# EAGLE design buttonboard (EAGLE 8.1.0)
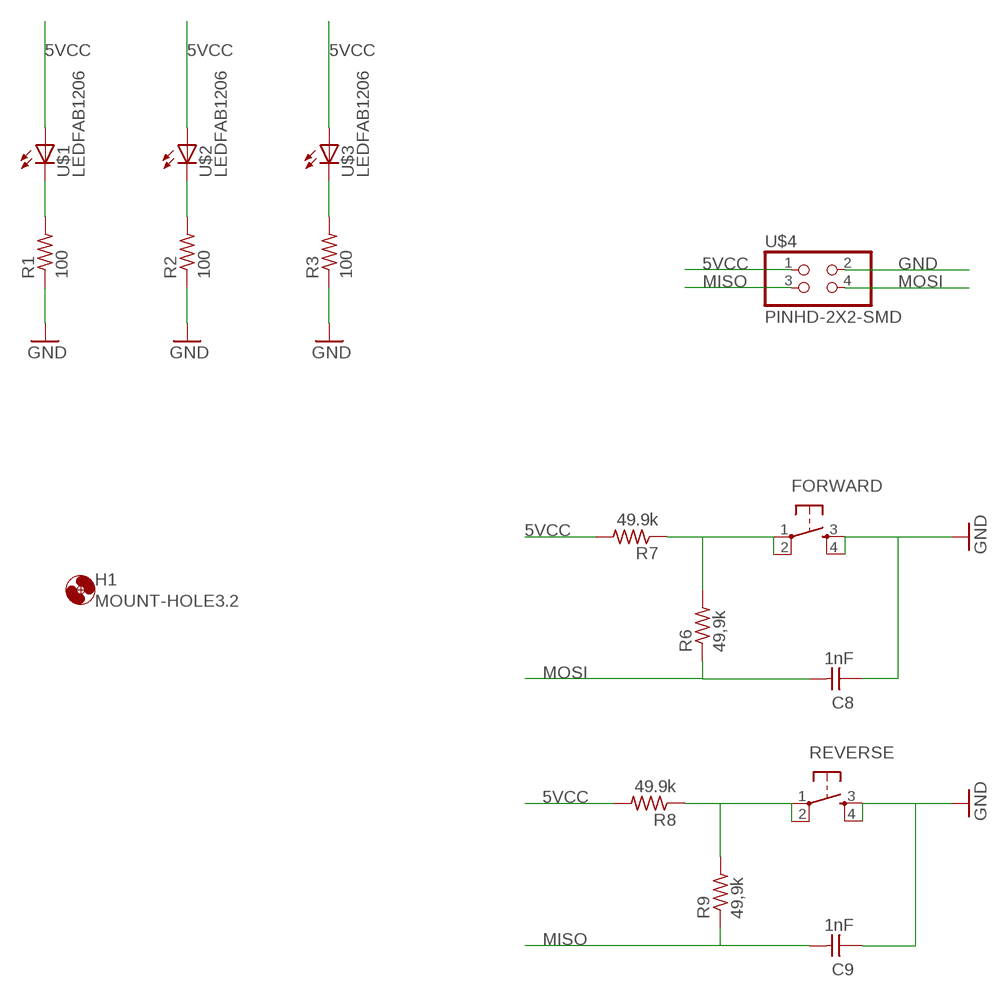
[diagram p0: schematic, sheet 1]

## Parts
C8  1nF  CAP-UNPOLARIZEDFAB  [C1206FAB]
C9  1nF  CAP-UNPOLARIZEDFAB  [C1206FAB]
FORWARD  6MM_SWITCH6MM_SWITCH  [6MM_SWITCH]
H1  MOUNT-HOLE3.2  [3,2]
R1  100  RES-US1206FAB  [R1206FAB]
R2  100  RES-US1206FAB  [R1206FAB]
R3  100  RES-US1206FAB  [R1206FAB]
R6  49,9k  RES-US1206FAB  [R1206FAB]
R7  49.9k  RES-US1206FAB  [R1206FAB]
R8  49.9k  RES-US1206FAB  [R1206FAB]
R9  49,9k  RES-US1206FAB  [R1206FAB]
REVERSE  6MM_SWITCH6MM_SWITCH  [6MM_SWITCH]
U$1  LEDFAB1206  [LED1206FAB]
U$2  LEDFAB1206  [LED1206FAB]
U$3  LEDFAB1206  [LED1206FAB]
U$4  PINHD-2X2-SMD  [2X02SMD]

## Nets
5VCC: R7.2 R8.2 U$1.1(A) U$2.1(A) U$3.1(A) U$4.1
GND: C8.1 C9.1 FORWARD.3(S) FORWARD.4(S1) R1.1 R2.1 R3.1 REVERSE.3(S) REVERSE.4(S1) U$4.2
MISO: C9.2 R9.1 U$4.3
MOSI: C8.2 R6.1 U$4.4
N$1: R1.2 U$1.2(C)
N$2: R2.2 U$2.2(C)
N$3: FORWARD.1(P) FORWARD.2(P1) R6.2 R7.1
N$4: R8.1 R9.2 REVERSE.1(P) REVERSE.2(P1)
N$5: R3.2 U$3.2(C)

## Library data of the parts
C8 C9 = fab:CAP-UNPOLARIZED
FORWARD REVERSE = fab:6MM_SWITCH: OMRON SWITCH
H1 = holes:MOUNT-HOLE: MOUNTING HOLE with drill center marker
R1-R3 R6-R9 = fab:RES-US: Resistor (US Symbol)
U$1-U$3 = fab:LED: LED
U$4 = fab:PINHD-2X2-SMD

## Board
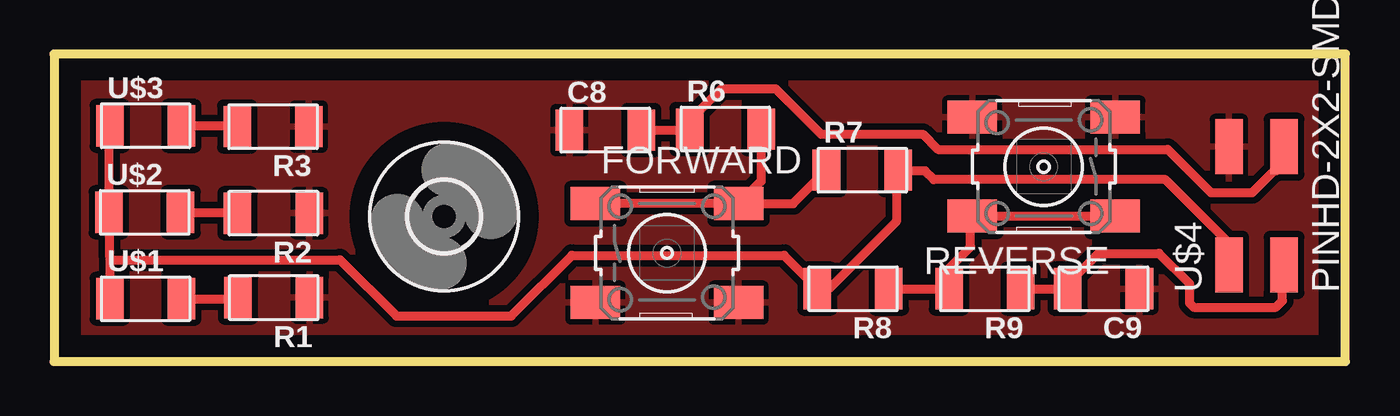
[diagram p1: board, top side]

Size 59.6 x 14.2 mm. Coordinates in mm from the lower left corner, seen from the top.
Outline: 0,0 59.6,0 59.6,14.2 0,14.2 0,0
Copper layers (1*16): Top 0.035mm / dielectric 1.5mm / Bottom 0.035mm
Design rules "default": minimum track width 10mil, minimum drill 24mil, track to track 8mil, track to pad 8mil, pad to pad 8mil, via to via 8mil, smd to smd 8mil, copper to edge 40mil, drill to drill 8mil, minimum pad ring 10mil, minimum via ring 8mil, stop-mask expansion 4mil, vias tented up to drill 0mil, thermal gap 10mil

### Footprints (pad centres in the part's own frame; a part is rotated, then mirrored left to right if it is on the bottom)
C1206FAB = smd 1.27 x 1.905: 1 -1.651,0; 2 1.651,0
6MM_SWITCH = smd 2.286 x 1.524: 1 -3.302,2.286; 2 3.302,2.286; 3 -3.302,-2.286; 4 3.302,-2.286
3,2 = hole 3.2: 0,0
R1206FAB = smd 1.27 x 1.905: 1 -1.651,0; 2 1.651,0
LED1206FAB = smd 1.27 x 1.905: 1 -1.651,0; 2 1.651,0
2X02SMD = smd 2.54 x 1.27: 1 -2.54,1.27; 2 2.92,1.27; 3 -2.54,-1.27; 4 2.92,-1.27

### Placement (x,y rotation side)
C8  25.44,10.69 0 top
C9  48.44,3.36 180 top
FORWARD  28.29,5.01 0 top
H1  18,6.7 0 top
R1  10.14,2.95 180 top
R2  10.12,6.85 180 top
R3  10.1,10.85 180 top
R6  30.98,10.74 0 top
R7  37.3,8.84 0 top
R8  36.88,3.36 180 top
R9  42.96,3.36 180 top
REVERSE  45.68,9 180 top
U$1  4.22,2.9 0 top
U$2  4.18,6.89 0 top
U$3  4.22,10.89 0 top
U$4  55.5,7 90 top

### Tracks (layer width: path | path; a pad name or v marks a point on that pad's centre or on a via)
5VCC
  Top 0.254: U$1.1 2.76,2.93 | 2.76,6.81 U$2.1 2.76,7.04 | 2.76,10.7 U$3.1
  Top 0.406: U$3.1 2.53,10.89 U$2.1 2.57,6.89 2.57,4.8 | 2.57,4.8 U$1.1 | U$4.1 54.23,5.47 51.3,8.4 40.6,8.4 40.2,8.8 38.99,8.8 R7.2 38.9,8.79 38.9,6.5 35.76,3.36 R8.2 33.69,4.9 23.9,4.9 21.1,2.1 15.8,2.1 13.2,4.7 2.67,4.7 2.57,4.8
GND
  pour Top (isolate 0.305): 0,0 59.6,0 59.5,14.2 -0.1,14.2
MISO
  Top 0.406: R9.1 C9.2 46.79,3.59 48.2,5 51,5 52.4,3.6 52.4,2.7 52.6,2.5 56.4,2.5 56.7,2.8 56.7,4.39 U$4.3 56.8,4.43
MOSI
  Top 0.254: 27.27,10.7 C8.2 | 29.1,10.7 R6.1
  Top 0.305: 29.74,10.74 R6.1
  Top 0.406: C8.2 29.09,10.69 29.1,10.7 | R6.1 29.33,11.13 30.8,12.6 33.3,12.6 35.4,10.5 40.1,10.5 40.8,9.8 51.4,9.8 53.4,7.8 55.3,7.8 56.3,8.8 56.4,8.8 56.6,9 56.6,9.75 U$4.4
N$1
  Top 0.254: 5.96,2.93 U$1.2 | R1.2 8.47,2.93
  Top 0.406: U$1.2 8.49,2.9 R1.2
N$2
  Top 0.254: 5.96,7.04 U$2.2 | R2.2 8.24,7.04
  Top 0.406: U$2.2 8.47,6.89 R2.2
N$3
  Top 0.254: 25.22,7.27 FORWARD.1
  Top 0.406: FORWARD.2 FORWARD.1 | FORWARD.2 34.11,7.3 R7.1 | R6.2 32.63,8.34 FORWARD.2
N$4
  Top 0.254: 38.7,3.39 R8.1 | 41.22,3.39 R9.2
  Top 0.406: R8.1 R9.2 41.31,4.31 42.3,5.3 42.3,6.64 REVERSE.2 REVERSE.1
N$5
  Top 0.254: 5.96,10.93 U$3.2 | R3.2 8.24,10.93
  Top 0.406: U$3.2 8.45,10.89 R3.2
